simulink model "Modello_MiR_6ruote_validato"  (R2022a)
settings: Solver=VariableStepAuto  StartTime=0.0  StopTime=time_s(end,1)  RelTol=1e-3
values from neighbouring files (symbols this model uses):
  a = 0.250    (= 0.25)    [Modello_MiR_6ruote_validato_script.m]    (also in Modello_MiR_2ruote_script.m; Modello_MiR_6ruote_script.m; Modello_MiR_UR_script.m)
  a1 = 0.18265    [Modello_MiR_6ruote_validato_script.m]    (also in Modello_MiR_2ruote_script.m = deg2rad(5); Modello_MiR_6ruote_script.m = deg2rad(5); Modello_MiR_UR_script.m; UR_DHtable_e.m = 0)
  a2 = 0.40857    [Modello_MiR_6ruote_validato_script.m]    (also in Modello_MiR_2ruote_script.m = deg2rad(25); Modello_MiR_6ruote_script.m = deg2rad(25); Modello_MiR_UR_script.m; UR_DHtable_e.m = 612)
  Att_C1 = 0.01    [Modello_MiR_6ruote_validato_script.m]    (also in Modello_MiR_UR_script.m)
  Att_C2 = 0.01    [Modello_MiR_6ruote_validato_script.m]    (also in Modello_MiR_UR_script.m)
  Att_C5 = 0.01    [Modello_MiR_6ruote_validato_script.m]    (also in Modello_MiR_UR_script.m)
  Att_C6 = 0.01    [Modello_MiR_6ruote_validato_script.m]    (also in Modello_MiR_UR_script.m)
  b = 0.1875    [Modello_MiR_6ruote_validato_script.m]    (also in Modello_MiR_2ruote_script.m; Modello_MiR_6ruote_script.m; Modello_MiR_UR_script.m)
  b_caster = 0.07    [Modello_MiR_6ruote_validato_script.m]    (also in Modello_MiR_2ruote_script.m; Modello_MiR_6ruote_script.m; Modello_MiR_UR_script.m)
  bd = 0.205    [Modello_MiR_6ruote_validato_script.m]    (also in Modello_MiR_2ruote_script.m; Modello_MiR_6ruote_script.m; Modello_MiR_UR_script.m)
  F23fun = @(u) (mv*9.801/4)-(mv*h*u(5)+(mv*9.801/4)*(2*a-b_caster*(cos(u(1))+cos(u(2)))))/(4*a-b_caster*(cos(u(1))+cos(u(2)))+b_caster*(cos(u(3))+cos(u(4))))    [Modello_MiR_6ruote_validato_script.m]    (also in Modello_MiR_6ruote_script.m = @(u) (mv*9.801/4)-u(7))
  F43fun = @(u) (1/(2*bd))*(mv*u(6)*h+((mv*h*u(5)+(mv*9.801/4)*(2*a-b_caster*(cos(u(1))+cos(u(2)))))/(4*a-b_caster*(cos(u(1))+cos(u(2)))+b_caster*(cos(u(3))+cos(u(4)))))*(2*bd-b_caster*(sin(u(3))+sin(u(4))))+((mv*9.801/4)-(mv*h*u(5)+(mv*9.801/4)*(2*a-b_caster*(cos(u(1))+cos(u(2)))))/(4*a-b_caster*(cos(u(1))+cos(u(2)))+b_caster*(cos(u(3))+cos(u(4)))))*(2*bd-b_caster*(sin(u(1))+sin(u(2)))))    [Modello_MiR_6ruote_validato_script.m]    (also in Modello_MiR_6ruote_script.m = @(u) (1/(2*bd))*(mv*u(6)*h+u(7)*(2*bd-b_caster*(sin(u(3))+si)
  F63fun = @(u) (mv*h*u(5)+(mv*9.801/4)*(2*a-b_caster*(cos(u(1))+cos(u(2)))))/(4*a-b_caster*(cos(u(1))+cos(u(2)))+b_caster*(cos(u(3))+cos(u(4))))    [Modello_MiR_6ruote_validato_script.m]    (also in Modello_MiR_6ruote_script.m)
  f_c = 0.29564    [Modello_MiR_6ruote_validato_script.m]    (also in Modello_MiR_UR_script.m)
  f_d3 = 0.35846    [Modello_MiR_6ruote_validato_script.m]    (also in Modello_MiR_UR_script.m)
  f_d4 = 0.2333    [Modello_MiR_6ruote_validato_script.m]    (also in Modello_MiR_UR_script.m)
  fa_c = 0.27474    [Modello_MiR_6ruote_validato_script.m]    (also in Modello_MiR_UR_script.m)
  fa_d3 = 0.3694    [Modello_MiR_6ruote_validato_script.m]    (also in Modello_MiR_UR_script.m)
  fa_d4 = 0.28065    [Modello_MiR_6ruote_validato_script.m]    (also in Modello_MiR_UR_script.m)
  fm_fun = @(u) (u <= -am2 || u >= am2) * 0 + (u > -am2 && u <= -am1) * (- u* Mza/(am2 -am1) - Mza* am2/(am2 -am1)) +           + (u > -am1 && u <= am1) * (Mza * u / am1) + (u > am1 && u < am2) * (Mza * u /(am1 -am2) - Mza * am2 /(am1 - am2))    [Modello_MiR_6ruote_validato_script.m]    (also in Modello_MiR_6ruote_script.m = @(u) (u <= -am2 | u >= am2)*0 + (u > -am2 && u <= -am1)*(- u; Modello_MiR_UR_script.m)
  Icw_1 = 1/2 * mcw * rc^2    (= 0.002004225735)    [Modello_MiR_6ruote_validato_script.m]    (also in Modello_MiR_2ruote_script.m; Modello_MiR_6ruote_script.m; Modello_MiR_UR_script.m)
  Icw_2 = 1/12 * mcw * ec^2 + 1/4 * mcw * rc^2    (= 0.00104098243873)    [Modello_MiR_6ruote_validato_script.m]    (also in Modello_MiR_2ruote_script.m; Modello_MiR_6ruote_script.m; Modello_MiR_UR_script.m)
  Idw_1 = 1/2 * mdw * rd^2    (= 0.00551836278784)    [Modello_MiR_6ruote_validato_script.m]    (also in Modello_MiR_2ruote_script.m; Transfer_Function_Gol_Gcl.m = Inertia_vect(jj,1); Modello_MiR_6ruote_script.m; Modello_MiR_UR_script.m)
  iMax = 20.7*1.1    (= 22.77)    [Modello_MiR_6ruote_validato_script.m]    (also in Modello_MiR_2ruote_script.m; Modello_MiR_6ruote_script.m; Modello_MiR_UR_script.m)
  Iv = mv * (l^2 + w^2)  / 12    (= 8.95033333333)    [Modello_MiR_6ruote_validato_script.m]    (also in Modello_MiR_2ruote_script.m = 6.75343333333; Modello_MiR_6ruote_script.m = 6.75343333333; Modello_MiR_UR_script.m = 6.75343333333)
  Kc = 0.15    [Modello_MiR_6ruote_validato_script.m]    (also in Modello_MiR_2ruote_script.m; Modello_MiR_6ruote_script.m; Modello_MiR_UR_script.m)
  Ki_i = 1    [Modello_MiR_6ruote_validato_script.m]    (also in Modello_MiR_2ruote_script.m; Modello_MiR_6ruote_script.m; Modello_MiR_UR_script.m)
  Ki_v = 1    [Modello_MiR_6ruote_validato_script.m]    (also in Modello_MiR_2ruote_script.m; Modello_MiR_6ruote_script.m; Modello_MiR_UR_script.m)
  kk = 0.00005    (= 5e-05)    [Modello_MiR_6ruote_validato_script.m]    (also in Modello_MiR_2ruote_script.m; Modello_MiR_6ruote_script.m; Modello_MiR_UR_script.m)
  Kp_i = 5    [Modello_MiR_6ruote_validato_script.m]    (also in Modello_MiR_2ruote_script.m; Modello_MiR_6ruote_script.m; Modello_MiR_UR_script.m)
  Kp_v = 5    [Modello_MiR_6ruote_validato_script.m]    (also in Modello_MiR_2ruote_script.m; Modello_MiR_6ruote_script.m; Modello_MiR_UR_script.m)
  kv = 1.5e-6    (= 1.5e-06)    [Modello_MiR_6ruote_validato_script.m]    (also in Modello_MiR_2ruote_script.m; Modello_MiR_6ruote_script.m; Modello_MiR_UR_script.m)
  L = R * tauE    (= 0.00181134822805)    [Modello_MiR_6ruote_validato_script.m]    (also in Modello_MiR_2ruote_script.m; Modello_MiR_6ruote_script.m; Modello_MiR_UR_script.m)
  mcw = rc^2 * pi * ec * rhopoliu + 1    (= 1.02616357632)    [Modello_MiR_6ruote_validato_script.m]    (also in Modello_MiR_2ruote_script.m; Modello_MiR_6ruote_script.m; Modello_MiR_UR_script.m)
  mv = 110    [Modello_MiR_6ruote_validato_script.m]    (also in Modello_MiR_2ruote_script.m = 83; Modello_MiR_6ruote_script.m = 83; Modello_MiR_UR_script.m = 83)
  Phi1_start = psi_mir(1,1)    [Modello_MiR_6ruote_validato_script.m]    (also in Modello_MiR_UR_script.m)
  Phi2_start = psi_mir(1,1)    [Modello_MiR_6ruote_validato_script.m]    (also in Modello_MiR_UR_script.m)
  Phi5_start = psi_mir(1,1)    [Modello_MiR_6ruote_validato_script.m]    (also in Modello_MiR_UR_script.m)
  Phi6_start = psi_mir(1,1)    [Modello_MiR_6ruote_validato_script.m]    (also in Modello_MiR_UR_script.m)
  Psi_start = psi_mir(1,1)    [Modello_MiR_6ruote_validato_script.m]    (also in Modello_MiR_6ruote_script.m = 1.57079632679; Modello_MiR_UR_script.m)
  R = velMax * TorqueMax / (iMax)^2    (= 1.81134822805)    [Modello_MiR_6ruote_validato_script.m]    (also in Modello_MiR_2ruote_script.m; Modello_MiR_6ruote_script.m; Modello_MiR_UR_script.m)
  rap_rid = 10.167    [Modello_MiR_6ruote_validato_script.m]    (also in Modello_MiR_2ruote_script.m; Modello_MiR_6ruote_script.m; Modello_MiR_UR_script.m)
  rc = 0.125/2    (= 0.0625)    [Modello_MiR_6ruote_validato_script.m]    (also in Modello_MiR_2ruote_script.m; Modello_MiR_6ruote_script.m; Modello_MiR_UR_script.m)
  rd = 0.1    [Modello_MiR_6ruote_validato_script.m]    (also in Modello_MiR_2ruote_script.m; Modello_MiR_6ruote_script.m; Modello_MiR_UR_script.m)
  s1 = 0.18987    [Modello_MiR_6ruote_validato_script.m]    (also in Modello_MiR_2ruote_script.m = 0.2; Modello_MiR_6ruote_script.m = 0.2; Modello_MiR_UR_script.m)
  s2 = 0.99533    [Modello_MiR_6ruote_validato_script.m]    (also in Modello_MiR_2ruote_script.m = 0.8; Modello_MiR_6ruote_script.m = 0.8; Modello_MiR_UR_script.m)
  Sx = spline(x ,fl_fun(x),zx)    [Modello_MiR_6ruote_script.m]
  Sy = spline(x ,ft_fun(x),zy)    [Modello_MiR_6ruote_script.m]
  VaMax = Kc * velMax    (= 41.2443991527)    [Modello_MiR_6ruote_validato_script.m]    (also in Modello_MiR_2ruote_script.m; Modello_MiR_6ruote_script.m; Modello_MiR_UR_script.m)
  X_start = traj(1,1)    [Modello_MiR_6ruote_validato_script.m]    (also in Modello_MiR_2ruote_script.m = input('Inserire coordinata x iniziale'); Modello_MiR_6ruote_script.m = input('Inserire coordinata x iniziale'); Modello_MiR_UR_script.m)
  Y_start = traj(1,2)    [Modello_MiR_6ruote_validato_script.m]    (also in Modello_MiR_2ruote_script.m = input('Inserire coordinata y iniziale'); Modello_MiR_6ruote_script.m = input('Inserire coordinata y iniziale'); Modello_MiR_UR_script.m)
undefined symbols (not defined in the file or in its folder): z
libraries: slpidlib x4
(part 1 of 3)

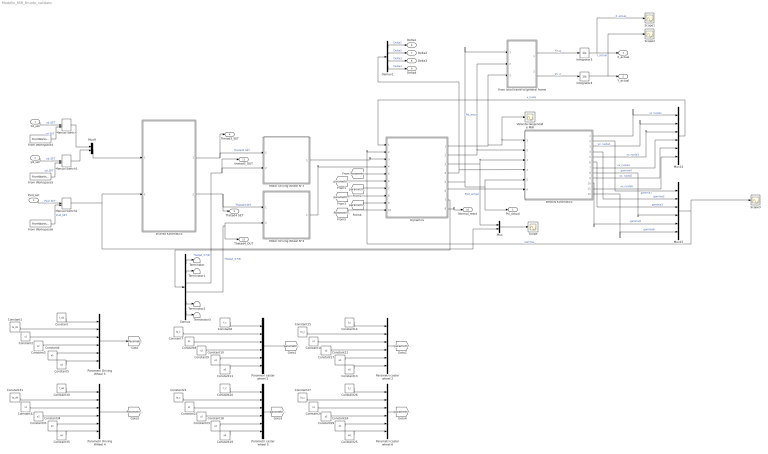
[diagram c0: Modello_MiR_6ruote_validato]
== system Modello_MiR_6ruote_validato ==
  xd_set : Inport
  yd_set : Inport  Port=2
  Psid_set : Inport  Port=3
  " Wheels Kinematics" : Subsystem
  Constant : Constant  Value=f_d3
  Constant1 : Constant  Value=fa_d3
  Constant{4,10,12,18,24,34} (6 alike) : Constant  Value=a1
  Constant{5,11,13,19,25,35} (6 alike) : Constant  Value=a2
  Constant{6,14,20,26} (4 alike) : Constant  Value=f_c
  Constant{7,15,21,27} (4 alike) : Constant  Value=fa_c
  Constant{2,8,16,22,28,32} (6 alike) : Constant  Value=s1
  Constant{3,9,17,23,29,33} (6 alike) : Constant  Value=s2
  Constant30 : Constant  Value=f_d4
  Constant31 : Constant  Value=fa_d4
  Demux : Demux  Outputs=6
  Demux1 : Demux
  Dynamics : Subsystem
  From Workspace4 : FromWorkspace  VariableName=[time_v xd_set]
  From Workspace5 : FromWorkspace  VariableName=[time_v yd_set]
  From Workspace6 : FromWorkspace  VariableName=[ time_v psid_set]
  From local frame to general frame : Subsystem
  Integrator3 : Integrator  InitialCondition=X_start
  Integrator4 : Integrator  InitialCondition=Y_start
  Inverse Kinematics : Subsystem
  Manual Switch : ManualSwitch  CurrentSetting=0
  Manual Switch1 : ManualSwitch  CurrentSetting=0
  Manual Switch2 : ManualSwitch  CurrentSetting=0
  Motor Driving Wheel N°3 : Subsystem
  Motor Driving Wheel N°4 : Subsystem
  Mux : Mux  Inputs=2
  Mux14 : Mux  Inputs=6
  Mux15 : Mux  Inputs=6
  Mux9 : Mux  Inputs=2
  Parametri Driving WHeel 4 : Mux  Inputs=6
  Parametri Driving Wheel 3 : Mux  Inputs=6
  "Parametri caster wheel 1 " : Mux  Inputs=6
  Parametri caster wheel 2 : Mux  Inputs=6
  Parametri caster wheel 5 : Mux  Inputs=6
  Parametri caster wheel 6 : Mux  Inputs=6
  Scope{,1..3} (4 alike) : Scope
  Terminator{,1..3} (4 alike) : Terminator
  Velocità tangenziale MIR : Scope
  Psi_actual : Outport
  Y_actual : Outport  Port=2
  X_actual : Outport  Port=3
  Thetad3_SET : Outport  Port=4
  Thetad4 SET : Outport  Port=5
  Delta1 : Outport  Port=6
  Delta2 : Outport  Port=7
  Delta3 : Outport  Port=8
  Delta4 : Outport  Port=9
  Normal_react : Outport  Port=10
  thetad3_OUT : Outport  Port=11
  Thetad4_OUT : Outport  Port=12
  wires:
  From local frame to general frame/2(Vy_g) -> Integrator4/1  "Vy_g"
  Dynamics/6(Phid) -> " Wheels Kinematics"/6(Phid)
  " Wheels Kinematics"/9(vx_ruota5) -> Mux14/5  "vx_ruota5"
  " Wheels Kinematics"/4(gamma2) -> Mux15/2  "gamma2"
  " Wheels Kinematics"/11(vx_ruota6) -> Mux14/6  "vx_ruota6"
  " Wheels Kinematics"/12(gamma6) -> Mux15/6  "gamma6"
  " Wheels Kinematics"/10(gamma5) -> Mux15/5  "gamma5"
  " Wheels Kinematics"/8(gamma4) -> Mux15/4  "gamma4"
  " Wheels Kinematics"/3(vx_ruota2) -> Mux14/2  "vx_ruota2"
  Dynamics/7(Thetad) -> Demux/1
  Motor Driving Wheel N°3/1(Cm_L) -> Dynamics/3(Cm3)
  From Workspace6/1 -> Manual Switch2/2  "Psid_SET"
  Mux/1 -> Scope/1
  Dynamics/4(Delta) -> Demux1/1, " Wheels Kinematics"/4(Delta)
  Dynamics/5(Psi) -> From local frame to general frame/1(Psi), Psi_actual/1, " Wheels Kinematics"/5(Psi)  "Psi_actual"
  " Wheels Kinematics"/7(vx_ruota4) -> Mux14/4  "vx_ruota4"
  Demux/6 -> Terminator3/1
  Mux15/1 -> Scope3/1, Dynamics/2(gamma)  "gamma"
  " Wheels Kinematics"/2(gamma1) -> Mux15/1  "gamma1"
  Demux/5 -> Terminator2/1
  Integrator4/1 -> Scope2/1, Y_actual/1  "Y_actual"
  Mux9/1 -> Inverse Kinematics/1(vSet)
  Dynamics/1(xd) -> From local frame to general frame/3(Vx), Velocità tangenziale MIR/1, " Wheels Kinematics"/1(xd)
  " Wheels Kinematics"/5(vx_ruota3) -> Mux14/3  "vx_ruota3"
  Dynamics/3(Psid) -> " Wheels Kinematics"/3(Psid), Mux/1  "Psid_actual"
  " Wheels Kinematics"/6(gamma3) -> Mux15/3  "gamma3"
  Integrator3/1 -> Scope1/1, X_actual/1  "X_actual"
  Inverse Kinematics/2(ThetaDotR) -> Thetad4 SET/1, Motor Driving Wheel N°4/1(ThetadR_SET)  "Thetad4 SET"
  Demux/4 -> Thetad4_OUT/1, Motor Driving Wheel N°4/2(ThetadR_FB)  "Thetad_4 F/B"
  Demux/2 -> Terminator1/1
  From local frame to general frame/1(Vx_g) -> Integrator3/1  "Vx_g"
  Mux14/1 -> Dynamics/1(vx_ruote)  "v_ruote"
  Dynamics/2(yd) -> From local frame to general frame/2(Vy), " Wheels Kinematics"/2(yd)
  Demux/1 -> Terminator/1
  " Wheels Kinematics"/1(vx_ruota1) -> Mux14/1  "vx_ruota1"
  Inverse Kinematics/1(ThetaDotL) -> Thetad3_SET/1, Motor Driving Wheel N°3/1(ThetadL_SET)  "Thetad3 SET"
  From Workspace5/1 -> Manual Switch1/2  "yd_SET"
  Motor Driving Wheel N°4/1(Cm_R) -> Dynamics/4(Cm4)
  Demux/3 -> thetad3_OUT/1, Motor Driving Wheel N°3/2(ThetadL_FB)  "Thetad_3 F/B"
  From Workspace4/1 -> Manual Switch/2  "xd_SET"
  Demux1/1 -> Delta1/1  "Delta1"
  Demux1/2 -> Delta2/1  "Delta2"
  Demux1/3 -> Delta3/1  "Delta3"
  Demux1/4 -> Delta4/1  "Delta4"
  Dynamics/8(Normal_react) -> Normal_react/1
  Parametri Driving Wheel 3/1 -> [Parametri]
  [Parametri] -> Dynamics/5(parametri_dw3)
  Constant/1 -> Parametri Driving Wheel 3/1
  Constant5/1 -> Parametri Driving Wheel 3/6
  Constant4/1 -> Parametri Driving Wheel 3/5
  Constant3/1 -> Parametri Driving Wheel 3/4
  Constant2/1 -> Parametri Driving Wheel 3/3
  Constant1/1 -> Parametri Driving Wheel 3/2
  xd_set/1 -> Manual Switch/1  "xd_SET"
  Manual Switch/1 -> Mux9/1
  yd_set/1 -> Manual Switch1/1  "yd_SET"
  Manual Switch1/1 -> Mux9/2
  Psid_set/1 -> Manual Switch2/1  "Psid_SET"
  Manual Switch2/1 -> Mux/2, Inverse Kinematics/2(psiDotSet)
  Constant10/1 -> "Parametri caster wheel 1 "/5
  Constant8/1 -> "Parametri caster wheel 1 "/3
  Constant9/1 -> "Parametri caster wheel 1 "/4
  Constant7/1 -> "Parametri caster wheel 1 "/2
  Constant11/1 -> "Parametri caster wheel 1 "/6
  Constant6/1 -> "Parametri caster wheel 1 "/1
  "Parametri caster wheel 1 "/1 -> [parametri_cw1]
  Constant12/1 -> Parametri caster wheel 2/5
  Constant17/1 -> Parametri caster wheel 2/4
  Constant16/1 -> Parametri caster wheel 2/3
  Constant13/1 -> Parametri caster wheel 2/6
  Constant15/1 -> Parametri caster wheel 2/2
  Constant14/1 -> Parametri caster wheel 2/1
  Parametri caster wheel 2/1 -> [parametri_cw2]
  Constant21/1 -> Parametri caster wheel 5/2
  Constant22/1 -> Parametri caster wheel 5/3
  Constant20/1 -> Parametri caster wheel 5/1
  Constant19/1 -> Parametri caster wheel 5/6
  Constant18/1 -> Parametri caster wheel 5/5
  Constant23/1 -> Parametri caster wheel 5/4
  Parametri caster wheel 5/1 -> [parametri_cw5]
  Constant27/1 -> Parametri caster wheel 6/2
  Constant28/1 -> Parametri caster wheel 6/3
  Constant26/1 -> Parametri caster wheel 6/1
  Constant25/1 -> Parametri caster wheel 6/6
  Constant24/1 -> Parametri caster wheel 6/5
  Constant29/1 -> Parametri caster wheel 6/4
  Parametri caster wheel 6/1 -> [parametri_cw6]
  [parametri_cw1] -> Dynamics/6(parametri_cw1)
  [parametri_cw2] -> Dynamics/7(parametri_cw2)
  [parametri_cw5] -> Dynamics/8(parametri_cw5)
  [parametri_cw6] -> Dynamics/9(parametri_cw6)
  Constant35/1 -> Parametri Driving WHeel 4/6
  Constant34/1 -> Parametri Driving WHeel 4/5
  Constant33/1 -> Parametri Driving WHeel 4/4
  Constant32/1 -> Parametri Driving WHeel 4/3
  Constant31/1 -> Parametri Driving WHeel 4/2
  Parametri Driving WHeel 4/1 -> [Parametri_dw4]
  Constant30/1 -> Parametri Driving WHeel 4/1
  [Parametri_dw4] -> Dynamics/10(parametri_dw4)

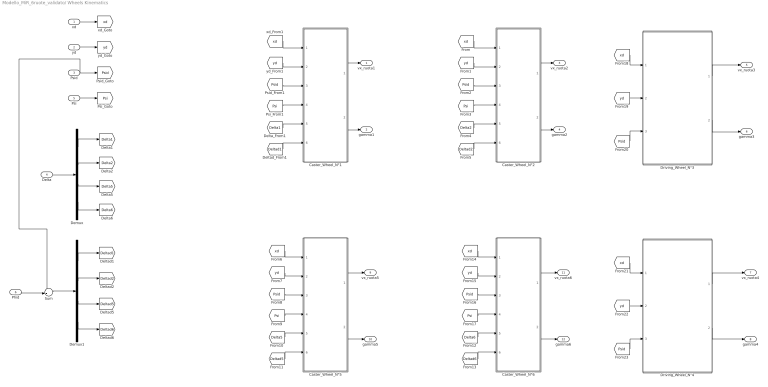
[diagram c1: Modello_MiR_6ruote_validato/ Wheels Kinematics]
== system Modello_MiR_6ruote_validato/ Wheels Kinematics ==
  xd : Inport
  yd : Inport  Port=2
  Psid : Inport  Port=3
  Delta : Inport  Port=4
  Psi : Inport  Port=5
  Phid : Inport  Port=6
  Caster_Wheel_N°1 : Subsystem
  Caster_Wheel_N°2 : Subsystem
  Caster_Wheel_N°5 : Subsystem
  Caster_Wheel_N°6 : Subsystem
  Demux : Demux
  Demux1 : Demux
  Driving_Wheel_N°3 : Subsystem
  Driving_Wheel_N°4 : Subsystem
  Sum : Sum  Inputs=-+|
  vx_ruota1 : Outport
  gamma1 : Outport  Port=2
  vx_ruota2 : Outport  Port=3
  gamma2 : Outport  Port=4
  vx_ruota3 : Outport  Port=5
  gamma3 : Outport  Port=6
  vx_ruota4 : Outport  Port=7
  gamma4 : Outport  Port=8
  vx_ruota5 : Outport  Port=9
  gamma5 : Outport  Port=10
  vx_ruota6 : Outport  Port=11
  gamma6 : Outport  Port=12
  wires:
  xd/1 -> [xd]
  yd/1 -> [yd]
  Psid/1 -> [Psid], Sum/1
  Delta/1 -> Demux/1
  Demux/1 -> [Delta1]
  Demux/2 -> [Delta2]
  Demux/3 -> [Delta5]
  Demux/4 -> [Delta6]
  Psi/1 -> [Psi]
  Phid/1 -> Sum/2
  Demux1/1 -> [Deltad1]
  Demux1/2 -> [Deltad2]
  Demux1/3 -> [Deltad5]
  Demux1/4 -> [Deltad6]
  [xd] -> Caster_Wheel_N°1/1(xd_From1)
  [yd] -> Caster_Wheel_N°1/2(yd_From1)
  [Psid] -> Caster_Wheel_N°1/3(Psid_From1)
  [Psi] -> Caster_Wheel_N°1/4(Psi_From1)
  [Delta1] -> Caster_Wheel_N°1/5(Delta_From1)
  [Deltad1] -> Caster_Wheel_N°1/6(Deltad_From1)
  Caster_Wheel_N°1/1(vx_ruota1) -> vx_ruota1/1
  Caster_Wheel_N°1/2(gamma1) -> gamma1/1
  [yd] -> Caster_Wheel_N°2/2(yd_From1)
  [Psi] -> Caster_Wheel_N°2/4(Psi_From1)
  [Psid] -> Caster_Wheel_N°2/3(Psid_From1)
  [xd] -> Caster_Wheel_N°2/1(xd_From1)
  [Deltad2] -> Caster_Wheel_N°2/6(Deltad_From2)
  Caster_Wheel_N°2/2(gamma2) -> gamma2/1
  [Delta2] -> Caster_Wheel_N°2/5(Delta_From2)
  Caster_Wheel_N°2/1(vx_ruota2) -> vx_ruota2/1
  [xd] -> Caster_Wheel_N°5/1(xd_From1)
  Caster_Wheel_N°5/2(gamma5) -> gamma5/1
  Caster_Wheel_N°5/1(vx_ruota5) -> vx_ruota5/1
  [Psid] -> Caster_Wheel_N°5/3(Psid_From1)
  [Deltad5] -> Caster_Wheel_N°5/6(Deltad_From5)
  [yd] -> Caster_Wheel_N°5/2(yd_From1)
  [Delta5] -> Caster_Wheel_N°5/5(Delta_From5)
  [Psi] -> Caster_Wheel_N°5/4(Psi_From1)
  Caster_Wheel_N°6/1(vx_ruota6) -> vx_ruota6/1
  [yd] -> Caster_Wheel_N°6/2(yd_From1)
  [Psid] -> Caster_Wheel_N°6/3(Psid_From1)
  [Psi] -> Caster_Wheel_N°6/4(Psi_From1)
  Caster_Wheel_N°6/2(gamma6) -> gamma6/1
  [xd] -> Caster_Wheel_N°6/1(xd_From1)
  [Delta6] -> Caster_Wheel_N°6/5(Delta_From6)
  [Deltad6] -> Caster_Wheel_N°6/6(Deltad_From6)
  [xd] -> Driving_Wheel_N°3/1(xd_From1)
  [yd] -> Driving_Wheel_N°3/2(yd_From1)
  [Psid] -> Driving_Wheel_N°3/3(Psid_From1)
  [xd] -> Driving_Wheel_N°4/1(xd_From1)
  [yd] -> Driving_Wheel_N°4/2(yd_From1)
  [Psid] -> Driving_Wheel_N°4/3(Psid_From1)
  Driving_Wheel_N°3/1(vx_ruota3) -> vx_ruota3/1
  Driving_Wheel_N°3/2(gamma3) -> gamma3/1
  Driving_Wheel_N°4/1(vx_ruota4) -> vx_ruota4/1
  Driving_Wheel_N°4/2(gamma4) -> gamma4/1
  Sum/1 -> Demux1/1

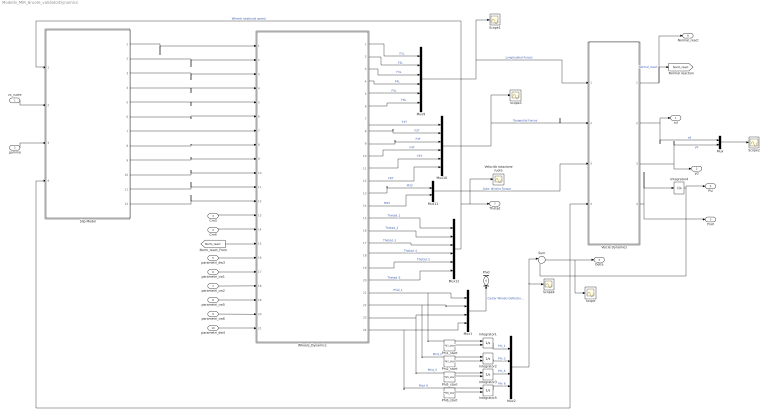
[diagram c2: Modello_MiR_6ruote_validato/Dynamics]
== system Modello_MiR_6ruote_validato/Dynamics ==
  vx_ruote : Inport
  gamma : Inport  Port=2
  Cm3 : Inport  Port=3
  Cm4 : Inport  Port=4
  parametri_dw3 : Inport  Port=5
  parametri_cw1 : Inport  Port=6
  parametri_cw2 : Inport  Port=7
  parametri_cw5 : Inport  Port=8
  parametri_cw6 : Inport  Port=9
  parametri_dw4 : Inport  Port=10
  Integrator{1..3,5} (4 alike) : Integrator  InitialConditionSource=external
  Integrator4 : Integrator  InitialCondition=Psi_start
  Mux : Mux  Inputs=2
  Mux1 : Mux
  Mux10 : Mux  Inputs=6
  Mux11 : Mux  Inputs=2
  Mux12 : Mux  Inputs=6
  Mux2 : Mux
  Mux9 : Mux  Inputs=6
  Phi1_start : Constant  Value=Phi1_start
  Phi2_start : Constant  Value=Phi2_start
  Phi5_start : Constant  Value=Phi5_start
  Phi6_start : Constant  Value=Phi6_start
  Scope{,1..4} (5 alike) : Scope
  Slip Model : Subsystem
  Sum : Sum  Inputs=|+-
  Veicle Dynamics : Subsystem
  Velocità rotazione ruote : Scope
  Wheels_Dynamics : Subsystem
  xd : Outport  PortDimensions=1
  yd : Outport  Port=2  PortDimensions=1
  Psid : Outport  Port=3  PortDimensions=1
  Delta : Outport  Port=4
  Psi : Outport  Port=5  PortDimensions=1
  Phid : Outport  Port=6
  Thetad : Outport  Port=7
  Normal_react : Outport  Port=8
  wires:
  Wheels_Dynamics/14(M43) -> Mux11/2  "M43"
  Wheels_Dynamics/23(Phid_5) -> Integrator3/1, Mux1/3  "Phid_5"
  Wheels_Dynamics/8(F2T) -> Mux10/2  "F2T"
  Wheels_Dynamics/12(F6T) -> Mux10/6  "F6T"
  Wheels_Dynamics/19(Thetad_5) -> Mux12/5  "Thetad_5"
  Wheels_Dynamics/18(Thetad_4) -> Mux12/4  "Thetad_4"
  Slip Model/1(Sigma1) -> Wheels_Dynamics/1(Sigma1)
  Wheels_Dynamics/2(F2L) -> Mux9/2  "F2L"
  Wheels_Dynamics/4(F4L) -> Mux9/4  "F4L"
  Wheels_Dynamics/3(F3L) -> Mux9/3  "F3L"
  Veicle Dynamics/4(Psid) -> Psid/1, Integrator4/1
  Wheels_Dynamics/1(F1L) -> Mux9/1  "F1L"
  Slip Model/3(Sigma3) -> Wheels_Dynamics/3(Sigma3)
  Slip Model/11(alpha5) -> Wheels_Dynamics/11(alpha5)
  Wheels_Dynamics/5(F5L) -> Mux9/5  "F5L"
  Slip Model/9(alpha3) -> Wheels_Dynamics/9(alpha3)
  Wheels_Dynamics/16(Thetad_2) -> Mux12/2  "Thetad_2"
  Mux1/1 -> Phid/1  "Caster Wheels Deflection Velocity"
  Cm3/1 -> Wheels_Dynamics/13(Cm3)
  Mux11/1 -> Veicle Dynamics/3(M)  "Auto_allining Torque"
  Wheels_Dynamics/10(F4T) -> Mux10/4  "F4T"
  Wheels_Dynamics/13(M33) -> Mux11/1  "M33"
  Mux12/1 -> Slip Model/1(Thetad_ruote), Velocità rotazione ruote/1, Thetad/1  "Wheels rotational speed"
  Mux10/1 -> Scope3/1, Veicle Dynamics/2(FT)  "Tangential Forces"
  Slip Model/5(Sigma5) -> Wheels_Dynamics/5(Sigma5)
  Wheels_Dynamics/21(Phid_1) -> Integrator1/1, Mux1/1  "Phid_1"
  Wheels_Dynamics/6(F6L) -> Mux9/6  "F6L"
  Wheels_Dynamics/17(Thetad_3) -> Mux12/3  "Thetad_3"
  Wheels_Dynamics/15(Thetad_1) -> Mux12/1  "Thetad_1"
  Wheels_Dynamics/24(Phid_6) -> Integrator5/1, Mux1/4  "Phid_6"
  Wheels_Dynamics/11(F5T) -> Mux10/5  "F5T"
  Wheels_Dynamics/9(F3T) -> Mux10/3  "F3T"
  Wheels_Dynamics/7(F1T) -> Mux10/1  "F1T"
  Wheels_Dynamics/22(Phid_2) -> Integrator2/1, Mux1/2  "Phid_2"
  Veicle Dynamics/1(Normal_react) -> Normal_react/1, [Norm_react]  "Normal_react"
  Veicle Dynamics/2(xd) -> Mux/1, xd/1  "xd"
  Mux2/1 -> Sum/1, Scope4/1
  Wheels_Dynamics/20(Thetad_6) -> Mux12/6  "Thetad_6"
  Slip Model/8(alpha2) -> Wheels_Dynamics/8(alpha2)
  Integrator4/1 -> Psi/1, Sum/2
  [Norm_react] -> Wheels_Dynamics/15(Normal_React)
  Veicle Dynamics/3(yd) -> Mux/2, yd/1  "yd"
  Mux9/1 -> Scope1/1, Veicle Dynamics/1(FL)  "Longitudinal Forces"
  Slip Model/4(Sigma4) -> Wheels_Dynamics/4(Sigma4)
  Slip Model/10(alpha4) -> Wheels_Dynamics/10(alpha4)
  Slip Model/12(alpha6) -> Wheels_Dynamics/12(alpha6)
  Slip Model/7(alpha1) -> Wheels_Dynamics/7(alpha1)
  Slip Model/2(Sigma2) -> Wheels_Dynamics/2(Sigma2)
  Slip Model/6(Sigma6) -> Wheels_Dynamics/6(Sigma6)
  vx_ruote/1 -> Slip Model/2(vx_ruote)
  gamma/1 -> Slip Model/3(gamma)
  Cm4/1 -> Wheels_Dynamics/14(Cm4)
  Mux/1 -> Scope2/1
  Sum/1 -> Slip Model/4(Delta), Scope/1, Delta/1, Veicle Dynamics/4(Delta)
  parametri_dw3/1 -> Wheels_Dynamics/16(parametri_dw3)
  parametri_cw1/1 -> Wheels_Dynamics/17(parametri_cw1)
  parametri_cw2/1 -> Wheels_Dynamics/18(parametri_cw2)
  parametri_cw5/1 -> Wheels_Dynamics/19(parametri_cw5)
  parametri_cw6/1 -> Wheels_Dynamics/20(parametri_cw6)
  Integrator1/1 -> Mux2/1  "Phi_1"
  Integrator2/1 -> Mux2/2  "Phi_2"
  Integrator3/1 -> Mux2/3  "Phi_5"
  Integrator5/1 -> Mux2/4  "Phi_6"
  Phi1_start/1 -> Integrator1/2
  Phi2_start/1 -> Integrator2/2
  Phi5_start/1 -> Integrator3/2
  Phi6_start/1 -> Integrator5/2
  parametri_dw4/1 -> Wheels_Dynamics/21(parametri_dw4)

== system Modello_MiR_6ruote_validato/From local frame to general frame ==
  Psi : Inport
  Vy : Inport  Port=2
  Vx : Inport  Port=3
  Cos : Trigonometry  Operator=cos
  Product{,1..3} (4 alike) : Product
  Sin : Trigonometry
  Sum : Sum  Inputs=-+
  Sum1 : Sum  Inputs=|++
  Vx_g : Outport
  Vy_g : Outport  Port=2
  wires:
  Product/1 -> Sum/2
  Sin/1 -> Product2/2, Product1/2
  Product1/1 -> Sum/1
  Vx/1 -> Product2/1, Product/1
  Product2/1 -> Sum1/1
  Cos/1 -> Product3/1, Product/2
  Product3/1 -> Sum1/2
  Psi/1 -> Sin/1, Cos/1
  Vy/1 -> Product3/2, Product1/1
  Sum/1 -> Vx_g/1
  Sum1/1 -> Vy_g/1

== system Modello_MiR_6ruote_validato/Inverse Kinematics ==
  vSet : Inport
  psiDotSet : Inport  Port=2
  Demux : Demux  Outputs=2
  MATLAB Function : MATLAB Function  TreatAsAtomicUnit=on
  MATLAB Function1 : MATLAB Function  TreatAsAtomicUnit=on
  Scope1 : Scope
  Scope2 : Scope
  Terminator : Terminator
  ThetaDotL : Outport
  ThetaDotR : Outport  Port=2
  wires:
  vSet/1 -> Demux/1
  Demux/1 -> MATLAB Function1/1(xd_set), MATLAB Function/1(xd_set)  "xd_set"
  psiDotSet/1 -> MATLAB Function1/2(psid_set), MATLAB Function/2(psid_set)
  MATLAB Function/1(Thetad_DR_SET) -> Scope1/1, ThetaDotR/1
  MATLAB Function1/1(Thetad_DL_SET) -> Scope2/1, ThetaDotL/1
  Demux/2 -> Terminator/1  "yd_set"

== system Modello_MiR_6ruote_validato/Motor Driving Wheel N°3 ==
  ThetadL_SET : Inport
  ThetadL_FB : Inport  Port=2
  Gain : Gain  Gain=rap_rid
  Gain1 : Gain  Gain=rap_rid
  Subsystem : Subsystem
  Subsystem1 : Subsystem
  Cm_L : Outport
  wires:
  Subsystem/1(VaRif) -> Subsystem1/1(VaRif)
  Subsystem1/2(iFB) -> Subsystem/3(iFB)
  ThetadL_SET/1 -> Gain1/1
  ThetadL_FB/1 -> Gain/1
  Subsystem1/1(Torque Cm) -> Cm_L/1
  Gain/1 -> Subsystem1/2(Thetad_FB), Subsystem/2(Thetad_FB)
  Gain1/1 -> Subsystem/1(Thetad_SET)

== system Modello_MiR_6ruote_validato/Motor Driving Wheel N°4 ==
  ThetadR_SET : Inport
  ThetadR_FB : Inport  Port=2
  Gain : Gain  Gain=rap_rid
  Gain1 : Gain  Gain=rap_rid
  Subsystem : Subsystem
  Subsystem1 : Subsystem
  Cm_R : Outport
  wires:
  Subsystem1/2(iFB) -> Subsystem/3(iFB)
  ThetadR_SET/1 -> Gain1/1
  Subsystem/1(VaRif) -> Subsystem1/1(VaRif)
  ThetadR_FB/1 -> Gain/1
  Subsystem1/1(Torque Cm) -> Cm_R/1
  Gain/1 -> Subsystem1/2(Thetad_FB), Subsystem/2(Thetad_FB)
  Gain1/1 -> Subsystem/1(Thetad_SET)

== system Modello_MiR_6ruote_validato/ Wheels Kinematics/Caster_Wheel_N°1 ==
  xd_From1 : Inport
  yd_From1 : Inport  Port=2
  Psid_From1 : Inport  Port=3
  Psi_From1 : Inport  Port=4
  Delta_From1 : Inport  Port=5
  Deltad_From1 : Inport  Port=6
  Interpreted MATLAB Function : MATLABFcn  MATLABFcn=(u(1)^2+u(2)^2)^0.5
  Interpreted MATLAB Function2 : MATLABFcn  MATLABFcn=asin(u(2)/((u(1)^2+u(2)^2)^0.5+(1/cccc)*((u(1)^2+u(2)^2)==0)))
  Mux : Mux  Inputs=6
  Mux1 : Mux  Inputs=2
  xd_ruota1 : MATLABFcn  MATLABFcn=(u(6)+u(3))*b_caster*sin(u(5))+u(1)-u(3)*b
  yd_ruota1 : MATLABFcn  MATLABFcn=-(u(6)+u(3))*b_caster*cos(u(5))+u(2)+u(3)*a
  vx_ruota1 : Outport  PortDimensions=1
  gamma1 : Outport  Port=2  PortDimensions=1
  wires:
  Mux/1 -> xd_ruota1/1, yd_ruota1/1
  Mux1/1 -> Interpreted MATLAB Function/1, Interpreted MATLAB Function2/1
  yd_ruota1/1 -> Mux1/2  "yd_ruota1"
  yd_From1/1 -> Mux/2
  xd_ruota1/1 -> Mux1/1  "xd_ruota1"
  xd_From1/1 -> Mux/1
  Psid_From1/1 -> Mux/3
  Delta_From1/1 -> Mux/5
  Psi_From1/1 -> Mux/4
  Deltad_From1/1 -> Mux/6
  Interpreted MATLAB Function2/1 -> gamma1/1  "gamma1"
  Interpreted MATLAB Function/1 -> vx_ruota1/1  "vx_ruota1"

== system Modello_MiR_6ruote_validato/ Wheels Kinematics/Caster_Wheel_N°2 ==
  xd_From1 : Inport
  yd_From1 : Inport  Port=2
  Psid_From1 : Inport  Port=3
  Psi_From1 : Inport  Port=4
  Delta_From2 : Inport  Port=5
  Deltad_From2 : Inport  Port=6
  Interpreted MATLAB Function : MATLABFcn  MATLABFcn=(u(1)^2+u(2)^2)^0.5
  Interpreted MATLAB Function2 : MATLABFcn  MATLABFcn=asin(u(2)/((u(1)^2+u(2)^2)^0.5+(1/cccc)*((u(1)^2+u(2)^2)==0)))
  Mux : Mux  Inputs=6
  Mux1 : Mux  Inputs=2
  xd_ruota2 : MATLABFcn  MATLABFcn=(u(6)+u(3))*b_caster*sin(u(5))+u(1)+u(3)*b
  yd_ruota2 : MATLABFcn  MATLABFcn=-(u(6)+u(3))*b_caster*cos(u(5))+u(2)+u(3)*a
  vx_ruota2 : Outport  PortDimensions=1
  gamma2 : Outport  Port=2  PortDimensions=1
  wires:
  Mux/1 -> xd_ruota2/1, yd_ruota2/1
  Mux1/1 -> Interpreted MATLAB Function/1, Interpreted MATLAB Function2/1
  yd_ruota2/1 -> Mux1/2  "yd_ruota2"
  yd_From1/1 -> Mux/2
  xd_ruota2/1 -> Mux1/1  "xd_ruota2"
  xd_From1/1 -> Mux/1
  Psid_From1/1 -> Mux/3
  Delta_From2/1 -> Mux/5
  Psi_From1/1 -> Mux/4
  Deltad_From2/1 -> Mux/6
  Interpreted MATLAB Function2/1 -> gamma2/1  "gamma2"
  Interpreted MATLAB Function/1 -> vx_ruota2/1  "vx_ruota2"

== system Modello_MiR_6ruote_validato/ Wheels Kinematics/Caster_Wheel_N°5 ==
  xd_From1 : Inport
  yd_From1 : Inport  Port=2
  Psid_From1 : Inport  Port=3
  Psi_From1 : Inport  Port=4
  Delta_From5 : Inport  Port=5
  Deltad_From5 : Inport  Port=6
  Interpreted MATLAB Function : MATLABFcn  MATLABFcn=(u(1)^2+u(2)^2)^0.5
  Interpreted MATLAB Function2 : MATLABFcn  MATLABFcn=asin(u(2)/((u(1)^2+u(2)^2)^0.5+(1/cccc)*((u(1)^2+u(2)^2)==0)))
  Mux : Mux  Inputs=6
  Mux1 : Mux  Inputs=2
  xd_ruota5 : MATLABFcn  MATLABFcn=(u(6)+u(3))*b_caster*sin(u(5))+u(1)-u(3)*b
  yd_ruota5 : MATLABFcn  MATLABFcn=-(u(6)+u(3))*b_caster*cos(u(5))+u(2)-u(3)*a
  vx_ruota5 : Outport  PortDimensions=1
  gamma5 : Outport  Port=2  PortDimensions=1
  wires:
  Mux/1 -> xd_ruota5/1, yd_ruota5/1
  Mux1/1 -> Interpreted MATLAB Function/1, Interpreted MATLAB Function2/1
  yd_ruota5/1 -> Mux1/2  "yd_ruota5"
  yd_From1/1 -> Mux/2
  xd_ruota5/1 -> Mux1/1  "xd_ruota5"
  xd_From1/1 -> Mux/1
  Psid_From1/1 -> Mux/3
  Delta_From5/1 -> Mux/5
  Psi_From1/1 -> Mux/4
  Deltad_From5/1 -> Mux/6
  Interpreted MATLAB Function2/1 -> gamma5/1  "gamma5"
  Interpreted MATLAB Function/1 -> vx_ruota5/1  "v_ruota5"

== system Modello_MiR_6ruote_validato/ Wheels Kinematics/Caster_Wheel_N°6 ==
  xd_From1 : Inport
  yd_From1 : Inport  Port=2
  Psid_From1 : Inport  Port=3
  Psi_From1 : Inport  Port=4
  Delta_From6 : Inport  Port=5
  Deltad_From6 : Inport  Port=6
  Interpreted MATLAB Function : MATLABFcn  MATLABFcn=(u(1)^2+u(2)^2)^0.5
  Interpreted MATLAB Function2 : MATLABFcn  MATLABFcn=asin(u(2)/((u(1)^2+u(2)^2)^0.5+(1/cccc)*((u(1)^2+u(2)^2)==0)))
  Mux : Mux  Inputs=6
  Mux1 : Mux  Inputs=2
  xd_ruota6 : MATLABFcn  MATLABFcn=(u(6)+u(3))*b_caster*sin(u(5))+u(1)+u(3)*b
  yd_ruota6 : MATLABFcn  MATLABFcn=-(u(6)+u(3))*b_caster*cos(u(5))+u(2)-u(3)*a
  vx_ruota6 : Outport  PortDimensions=1
  gamma6 : Outport  Port=2  PortDimensions=1
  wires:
  Mux/1 -> xd_ruota6/1, yd_ruota6/1
  Mux1/1 -> Interpreted MATLAB Function/1, Interpreted MATLAB Function2/1
  yd_ruota6/1 -> Mux1/2  "yd_ruota6"
  yd_From1/1 -> Mux/2
  xd_ruota6/1 -> Mux1/1  "xd_ruota6"
  xd_From1/1 -> Mux/1
  Psid_From1/1 -> Mux/3
  Delta_From6/1 -> Mux/5
  Psi_From1/1 -> Mux/4
  Deltad_From6/1 -> Mux/6
  Interpreted MATLAB Function2/1 -> gamma6/1  "gamma6"
  Interpreted MATLAB Function/1 -> vx_ruota6/1  "v_ruota6"

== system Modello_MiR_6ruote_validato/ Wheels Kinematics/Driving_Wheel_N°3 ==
  xd_From1 : Inport
  yd_From1 : Inport  Port=2
  Psid_From1 : Inport  Port=3
  Interpreted MATLAB Function : MATLABFcn  MATLABFcn=u(1) - u(3)*bd
  Interpreted MATLAB Function1 : MATLABFcn  MATLABFcn=u(2)
  Interpreted MATLAB Function3 : MATLABFcn  MATLABFcn=asin(u(2)/((u(1)^2+u(2)^2)^0.5+(1/cccc)*((u(1)^2+u(2)^2)==0)))
  Mux : Mux  Inputs=3
  Mux1 : Mux  Inputs=2
  Scope1 : Scope
  vx_ruota3 : Outport  PortDimensions=1
  gamma3 : Outport  Port=2  PortDimensions=1
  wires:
  yd_From1/1 -> Mux/2
  xd_From1/1 -> Mux/1
  Psid_From1/1 -> Mux/3
  Mux/1 -> Interpreted MATLAB Function1/1, Interpreted MATLAB Function/1
  Interpreted MATLAB Function1/1 -> Mux1/2  "yd_ruota3"
  Interpreted MATLAB Function/1 -> vx_ruota3/1, Mux1/1  "xd_ruota3"
  Interpreted MATLAB Function3/1 -> gamma3/1  "gamma3"
  Mux1/1 -> Scope1/1, Interpreted MATLAB Function3/1

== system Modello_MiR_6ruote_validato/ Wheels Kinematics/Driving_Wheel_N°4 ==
  xd_From1 : Inport
  yd_From1 : Inport  Port=2
  Psid_From1 : Inport  Port=3
  Interpreted MATLAB Function : MATLABFcn  MATLABFcn=u(1) + u(3)*bd
  Interpreted MATLAB Function1 : MATLABFcn  MATLABFcn=u(2)
  Interpreted MATLAB Function3 : MATLABFcn  MATLABFcn=asin(u(2)/((u(1)^2+u(2)^2)^0.5+(1/cccc)*((u(1)^2+u(2)^2)==0)))
  Mux : Mux  Inputs=3
  Mux1 : Mux  Inputs=2
  Scope : Scope
  vx_ruota4 : Outport  PortDimensions=1
  gamma4 : Outport  Port=2  PortDimensions=1
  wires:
  yd_From1/1 -> Mux/2
  xd_From1/1 -> Mux/1
  Psid_From1/1 -> Mux/3
  Mux/1 -> Interpreted MATLAB Function1/1, Interpreted MATLAB Function/1
  Interpreted MATLAB Function1/1 -> Mux1/2  "yd_ruota4"
  Interpreted MATLAB Function/1 -> vx_ruota4/1, Mux1/1, Scope/1  "xd_ruota4"
  Mux1/1 -> Interpreted MATLAB Function3/1
  Interpreted MATLAB Function3/1 -> gamma4/1  "gamma4"

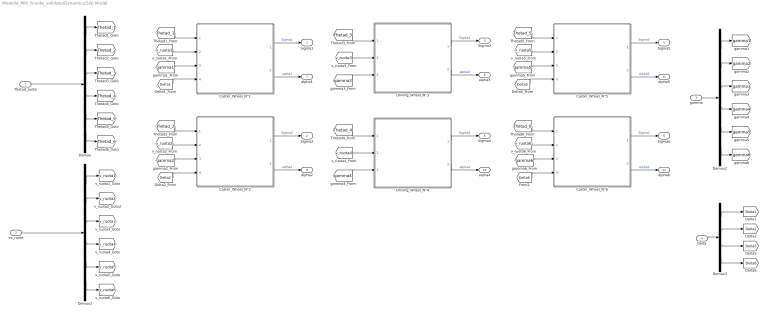
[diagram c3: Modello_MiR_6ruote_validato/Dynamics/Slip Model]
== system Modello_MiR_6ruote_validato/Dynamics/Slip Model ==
  Thetad_ruote : Inport
  vx_ruote : Inport  Port=2
  gamma : Inport  Port=3
  Delta : Inport  Port=4
  Caster_Wheel_N°1 : Subsystem
  Caster_Wheel_N°2 : Subsystem
  Caster_Wheel_N°5 : Subsystem
  Caster_Wheel_N°6 : Subsystem
  Demux : Demux  Outputs=6
  Demux1 : Demux  Outputs=6
  Demux2 : Demux  Outputs=6
  Demux3 : Demux
  Driving_Wheel_N°3 : Subsystem
  Driving_Wheel_N°4 : Subsystem
  Sigma1 : Outport  PortDimensions=1
  Sigma2 : Outport  Port=2  PortDimensions=1
  Sigma3 : Outport  Port=3  PortDimensions=1
  Sigma4 : Outport  Port=4  PortDimensions=1
  Sigma5 : Outport  Port=5  PortDimensions=1
  Sigma6 : Outport  Port=6  PortDimensions=1
  alpha1 : Outport  Port=7  PortDimensions=1
  alpha2 : Outport  Port=8  PortDimensions=1
  alpha3 : Outport  Port=9  PortDimensions=1
  alpha4 : Outport  Port=10  PortDimensions=1
  alpha5 : Outport  Port=11  PortDimensions=1
  alpha6 : Outport  Port=12  PortDimensions=1
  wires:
  Caster_Wheel_N°1/2(alpha1) -> alpha1/1  "alpha1"
  Demux/3 -> [Thetad_3]
  [Delta5] -> Caster_Wheel_N°5/4(Delta5)
  Demux1/1 -> [v_ruota1]
  Driving_Wheel_N°3/2(alpha3) -> alpha3/1  "alpha3"
  Demux1/6 -> [v_ruota6]
  Caster_Wheel_N°5/2(alpha5) -> alpha5/1  "alpha5"
  Demux1/2 -> [v_ruota2]
  Demux/1 -> [Thetad_1]
  Demux3/2 -> [Delta2]
  [v_ruota6] -> Caster_Wheel_N°6/2(vx_ruota6)
  Driving_Wheel_N°4/1(Sigma4) -> Sigma4/1  "Sigma4"
  Demux2/5 -> [gamma5]
  Caster_Wheel_N°6/2(alpha6) -> alpha6/1  "alpha2"
  Driving_Wheel_N°3/1(Sigma3) -> Sigma3/1  "Sigma3"
  [Thetad_1] -> Caster_Wheel_N°1/1(Thetad_1)
  Demux/2 -> [Thetad_2]
  Driving_Wheel_N°4/2(alpha4) -> alpha4/1  "alpha4"
  Demux1/4 -> [v_ruota4]
  Thetad_ruote/1 -> Demux/1
  [gamma6] -> Caster_Wheel_N°6/3(gamma6)
  Caster_Wheel_N°2/2(alpha2) -> alpha2/1  "alpha2"
  Caster_Wheel_N°5/1(Sigma5) -> Sigma5/1  "Sigma5"
  [v_ruota3] -> Driving_Wheel_N°3/2(vx_ruota3)
  Caster_Wheel_N°1/1(Sigma1) -> Sigma1/1  "Sigma1"
  [Thetad_4] -> Driving_Wheel_N°4/1(Thetad_4)
  Demux/5 -> [Thetad_5]
  Caster_Wheel_N°2/1(Sigma2) -> Sigma2/1  "Sigma2"
  [gamma1] -> Caster_Wheel_N°1/3(gamma1)
  Demux/4 -> [Thetad_4]
  [v_ruota4] -> Driving_Wheel_N°4/2(vx_ruota4)
  Demux3/1 -> [Delta1]
  Caster_Wheel_N°6/1(Sigma6) -> Sigma6/1  "Sigma2"
  Demux3/3 -> [Delta5]
  Demux/6 -> [Thetad_6]
  Demux2/6 -> [gamma6]
  [Thetad_5] -> Caster_Wheel_N°5/1(Thetad_5)
  [Delta1] -> Caster_Wheel_N°1/4(Delta1)
  Demux1/5 -> [v_ruota5]
  Delta/1 -> Demux3/1
  gamma/1 -> Demux2/1
  [Thetad_3] -> Driving_Wheel_N°3/1(Thetad_3)
  vx_ruote/1 -> Demux1/1
  Demux2/4 -> [gamma4]
  Demux2/1 -> [gamma1]
  Demux2/2 -> [gamma2]
  [v_ruota2] -> Caster_Wheel_N°2/2(vx_ruota2)
  [gamma5] -> Caster_Wheel_N°5/3(gamma5)
  Demux2/3 -> [gamma3]
  [gamma4] -> Driving_Wheel_N°4/3(gamma4)
  [Thetad_2] -> Caster_Wheel_N°2/1(Thetad_2)
  [v_ruota1] -> Caster_Wheel_N°1/2(vx_ruota1)
  [gamma2] -> Caster_Wheel_N°2/3(gamma2)
  Demux1/3 -> [v_ruota3]
  [Delta6] -> Caster_Wheel_N°6/4(Delta6)
  [Thetad_6] -> Caster_Wheel_N°6/1(Thetad_6)
  Demux3/4 -> [Delta6]
  [Delta2] -> Caster_Wheel_N°2/4(Delta2)
  [gamma3] -> Driving_Wheel_N°3/3(gamma3)
  [v_ruota5] -> Caster_Wheel_N°5/2(vx_ruota5)

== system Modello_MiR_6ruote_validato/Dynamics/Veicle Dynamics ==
  FL : Inport
  FT : Inport  Port=2
  M : Inport  Port=3
  Delta : Inport  Port=4
  Demux : Demux
  Integrator : Integrator
  Integrator1 : Integrator
  Integrator6 : Integrator
  Mux14 : Mux  Inputs=6
  Normal Reaction : Subsystem
  Rotation Dynamics : Subsystem
  Rotational Matrix : MATLAB Function  TreatAsAtomicUnit=on
  Scope : Scope
  Translation Dynamics : Subsystem
  Normal_react : Outport
  xd : Outport  Port=2  PortDimensions=1
  yd : Outport  Port=3  PortDimensions=1
  Psid : Outport  Port=4  PortDimensions=1
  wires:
  Normal Reaction/4(F43) -> Mux14/4  "F43"
  Demux/1 -> Normal Reaction/1(Delta1)
  Demux/2 -> Normal Reaction/2(Delta2)
  Normal Reaction/5(F53) -> Mux14/5  "F53"
  Demux/4 -> Normal Reaction/4(Delta6)
  Normal Reaction/1(F13) -> Mux14/1  "F13"
  Rotation Dynamics/1(Psidd) -> Integrator6/1
  Normal Reaction/2(F23) -> Mux14/2  "F23"
  Normal Reaction/6(F63) -> Mux14/6  "F63"
  Demux/3 -> Normal Reaction/3(Delta5)
  Normal Reaction/3(F33) -> Mux14/3  "F33"
  Integrator6/1 -> Psid/1, Translation Dynamics/5(Psid)  "Psid"
  Mux14/1 -> Scope/1, Normal_react/1
  Delta/1 -> Rotation Dynamics/2("Delta "), Demux/1, Rotational Matrix/3(Delta)
  Rotational Matrix/2(Fy_generalized) -> Rotation Dynamics/3(Fy_generalized), Translation Dynamics/2(Fy_generalized)
  FL/1 -> Rotational Matrix/1(FL)
  FT/1 -> Rotational Matrix/2(FT)
  Rotational Matrix/1(Fx_generalized) -> Rotation Dynamics/1(Fx_generalized), Translation Dynamics/1(Fx_generalized)
  Translation Dynamics/1(xdd) -> Integrator/1
  Translation Dynamics/2(ydd) -> Integrator1/1
  Integrator/1 -> Translation Dynamics/3(xd), xd/1
  Integrator1/1 -> Translation Dynamics/4(yd), yd/1
  M/1 -> Rotation Dynamics/4(M)
  Translation Dynamics/3(a_tau) -> Normal Reaction/5(a_tau)
  Translation Dynamics/4(a_n) -> Normal Reaction/6(a_n)

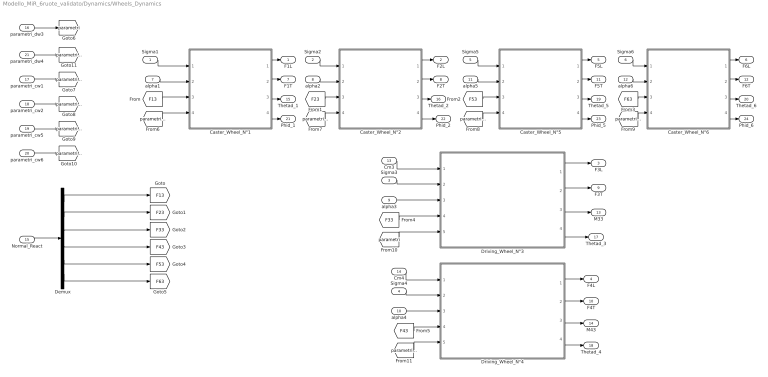
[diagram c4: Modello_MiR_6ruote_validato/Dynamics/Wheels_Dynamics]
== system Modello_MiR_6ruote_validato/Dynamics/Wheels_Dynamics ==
  Sigma1 : Inport
  Sigma2 : Inport  Port=2
  Sigma3 : Inport  Port=3
  Sigma4 : Inport  Port=4
  Sigma5 : Inport  Port=5
  Sigma6 : Inport  Port=6
  alpha1 : Inport  Port=7
  alpha2 : Inport  Port=8
  alpha3 : Inport  Port=9
  alpha4 : Inport  Port=10
  alpha5 : Inport  Port=11
  alpha6 : Inport  Port=12
  Cm3 : Inport  Port=13
  Cm4 : Inport  Port=14
  Normal_React : Inport  Port=15
  parametri_dw3 : Inport  Port=16
  parametri_cw1 : Inport  Port=17
  parametri_cw2 : Inport  Port=18
  parametri_cw5 : Inport  Port=19
  parametri_cw6 : Inport  Port=20
  parametri_dw4 : Inport  Port=21
  Caster_Wheel_N°1 : Subsystem
  Caster_Wheel_N°2 : Subsystem
  Caster_Wheel_N°5 : Subsystem
  Caster_Wheel_N°6 : Subsystem
  Demux : Demux  Outputs=6
  Driving_Wheel_N°3 : Subsystem
  Driving_Wheel_N°4 : Subsystem
  F1L : Outport  PortDimensions=1
  F2L : Outport  Port=2  PortDimensions=1
  F3L : Outport  Port=3  PortDimensions=1
  F4L : Outport  Port=4  PortDimensions=1
  F5L : Outport  Port=5  PortDimensions=1
  F6L : Outport  Port=6  PortDimensions=1
  F1T : Outport  Port=7  PortDimensions=1
  F2T : Outport  Port=8  PortDimensions=1
  F3T : Outport  Port=9  PortDimensions=1
  F4T : Outport  Port=10  PortDimensions=1
  F5T : Outport  Port=11  PortDimensions=1
  F6T : Outport  Port=12  PortDimensions=1
  M33 : Outport  Port=13  PortDimensions=1
  M43 : Outport  Port=14  PortDimensions=1
  Thetad_1 : Outport  Port=15  PortDimensions=1
  Thetad_2 : Outport  Port=16  PortDimensions=1
  Thetad_3 : Outport  Port=17  PortDimensions=1
  Thetad_4 : Outport  Port=18  PortDimensions=1
  Thetad_5 : Outport  Port=19  PortDimensions=1
  Thetad_6 : Outport  Port=20  PortDimensions=1
  Phid_1 : Outport  Port=21  PortDimensions=1
  Phid_2 : Outport  Port=22  PortDimensions=1
  Phid_5 : Outport  Port=23  PortDimensions=1
  Phid_6 : Outport  Port=24  PortDimensions=1
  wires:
  Sigma5/1 -> Caster_Wheel_N°5/1(Sigma5)
  Caster_Wheel_N°6/1(F6L) -> F6L/1
  Sigma2/1 -> Caster_Wheel_N°2/1(Sigma2)
  Caster_Wheel_N°6/3(Thetad_6) -> Thetad_6/1
  Caster_Wheel_N°2/1(F2L) -> F2L/1
  Caster_Wheel_N°6/4(Phid_6) -> Phid_6/1
  Caster_Wheel_N°5/3(Thetad_5) -> Thetad_5/1
  alpha1/1 -> Caster_Wheel_N°1/2(alpha1)
  Sigma1/1 -> Caster_Wheel_N°1/1(Sigma1)
  Caster_Wheel_N°1/2(F1T) -> F1T/1
  Caster_Wheel_N°1/4(Phid_1) -> Phid_1/1
  Caster_Wheel_N°5/2(F5T) -> F5T/1
  Caster_Wheel_N°5/4(Phid_5) -> Phid_5/1
  Caster_Wheel_N°5/1(F5L) -> F5L/1
  Caster_Wheel_N°6/2(F6T) -> F6T/1
  Sigma6/1 -> Caster_Wheel_N°6/1(Sigma6)
  alpha6/1 -> Caster_Wheel_N°6/2(alpha6)
  Caster_Wheel_N°2/4(Phid_2) -> Phid_2/1
  alpha5/1 -> Caster_Wheel_N°5/2(alpha5)
  Caster_Wheel_N°2/2(F2T) -> F2T/1
  Caster_Wheel_N°1/1(F1L) -> F1L/1
  alpha2/1 -> Caster_Wheel_N°2/2(alpha2)
  Caster_Wheel_N°2/3(Thetad_2) -> Thetad_2/1
  Caster_Wheel_N°1/3(Thetad_1) -> Thetad_1/1
  alpha4/1 -> Driving_Wheel_N°4/3(alpha4)
  alpha3/1 -> Driving_Wheel_N°3/3(alpha3)
  Driving_Wheel_N°4/2(F4T) -> F4T/1
  Driving_Wheel_N°3/3(M33) -> M33/1
  Driving_Wheel_N°4/4(Thetad_4) -> Thetad_4/1
  Sigma4/1 -> Driving_Wheel_N°4/2(Sigma4)
  Driving_Wheel_N°4/3(M43) -> M43/1
  Sigma3/1 -> Driving_Wheel_N°3/2(Sigma3)
  Driving_Wheel_N°3/1(F3L) -> F3L/1
  Cm3/1 -> Driving_Wheel_N°3/1(Cm3)
  Driving_Wheel_N°3/4(Thetad_3) -> Thetad_3/1
  Driving_Wheel_N°3/2(F3T) -> F3T/1
  Driving_Wheel_N°4/1(F4L) -> F4L/1
  Cm4/1 -> Driving_Wheel_N°4/1(Cm4)
  Normal_React/1 -> Demux/1
  [F13] -> Caster_Wheel_N°1/3(F13)
  [F23] -> Caster_Wheel_N°2/3(F23)
  [F53] -> Caster_Wheel_N°5/3(F53)
  [F63] -> Caster_Wheel_N°6/3(F63)
  [F33] -> Driving_Wheel_N°3/4(F33)
  [F43] -> Driving_Wheel_N°4/4(F43)
  Demux/1 -> [F13]
  Demux/2 -> [F23]
  Demux/3 -> [F33]
  Demux/4 -> [F43]
  Demux/5 -> [F53]
  Demux/6 -> [F63]
  parametri_dw3/1 -> [parametri]
  [parametri_cw1] -> Caster_Wheel_N°1/4(parametri_cw1)
  [parametri_cw2] -> Caster_Wheel_N°2/4(parametri)
  [parametri_cw5] -> Caster_Wheel_N°5/4(parametri)
  [parametri_cw6] -> Caster_Wheel_N°6/4(parametri)
  [parametri] -> Driving_Wheel_N°3/5(parametri_dw3)
  [parametri_dw4] -> Driving_Wheel_N°4/5(parametri_dw4)
  parametri_cw1/1 -> [parametri_cw1]
  parametri_cw2/1 -> [parametri_cw2]
  parametri_cw5/1 -> [parametri_cw5]
  parametri_cw6/1 -> [parametri_cw6]
  parametri_dw4/1 -> [parametri_dw4]

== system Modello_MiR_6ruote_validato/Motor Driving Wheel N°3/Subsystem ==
  Thetad_SET : Inport
  Thetad_FB : Inport  Port=2
  iFB : Inport  Port=3
  " 1" : slpidlib/PID Controller  Controller=PID  Form=Parallel  TimeDomain=Continuous-time  UseExternalTs=off  SampleTime=-1  IntegratorMethod=Forward Euler  FilterMethod=Forward Euler  ControllerParametersSource=internal  P=Kp_v  I=Ki_v  UseKiTs=off  D=0  N=1  UseFilter=on  TunerSelectOption=Transfer Function Based (PID Tuner App)  InitialConditionSource=internal  InitialConditionForIntegrator=0  InitialConditionForFilter=0  DifferentiatorICPrevScaledInput=0  ExternalReset=none  TrackingMode=off  Kt=1  LimitOutput=on  SatLimitsSource=internal  UpperSaturationLimit=iMax  LowerSaturationLimit=-iMax  LinearizeAsGain=on  AntiWindupMode=back-calculation  Kb=1  POutMin=[]  POutMax=[]  IOutMin=[]  IOutMax=[]  DOutMin=[]  DOutMax=[]  NOutMin=[]  NOutMax=[]  SumOutMin=[]  SumOutMax=[]  SaturationOutMin=[]  SaturationOutMax=[]  PParamMin=0  PParamMax=[]  IParamMin=0  IParamMax=[]  DParamMin=0  DParamMax=[]  NParamMin=[]  NParamMax=[]  KbParamMin=[]  KbParamMax=[]  KtParamMin=[]  KtParamMax=[]  KbOutMin=[]  KbOutMax=[]  KtOutMin=[]  KtOutMax=[]  IntegratorOutMin=[]  IntegratorOutMax=[]  FilterOutMin=[]  FilterOutMax=[]  SumI1OutMin=[]  SumI1OutMax=[]  SumI2OutMin=[]  SumI2OutMax=[]  SumI3OutMin=[]  SumI3OutMax=[]  SumI4OutMin=[]  SumI4OutMax=[]  SumDOutMin=[]  SumDOutMax=[]  DifferentiatorOutMin=[]  DifferentiatorOutMax=[]  FilterDiffOutCoefMin=[]  FilterDiffOutCoefMax=[]  ReciprocalOutMin=[]  ReciprocalOutMax=[]  SumDenOutMin=[]  SumDenOutMax=[]  SumNumOutMin=[]  SumNumOutMax=[]  DivideOutMin=[]  DivideOutMax=[]  UdiffTsProdOutMin=[]  UdiffTsProdOutMax=[]  NTsProdOutMin=[]  NTsProdOutMax=[]  UintegralTsProdOutMin=[]  UintegralTsProdOutMax=[]  UngainTsProdOutMin=[]  UngainTsProdOutMax=[]  IntegratorContinuousStateAttributes=''  IntegratorStateMustResolveToSignalObject=off  IntegratorRTWStateStorageClass=Auto  FilterContinuousStateAttributes=''  FilterStateMustResolveToSignalObject=off  FilterRTWStateStorageClass=Auto  ParallelPVariant=InternalParameters  IdealPVariant=Disabled  IVariant=InternalParameters  DVariant=InternalParameters  IntegratorVariant=Continuous  SatVariant=Enabled  AWVariant=BackCalculation  PCopyVariant=Disabled  TRVariant=Disabled  FdbkBlocksVariant=Forward  IdealPFdbkVariant=Disabled  SatFdbkVariant=Disabled  DerivativeFilterVariant=ContFilter  NVariant=InternalParameters  NCopyVariant=Disabled  FilterICVariant=InternalICsFilter  IntegratorICVariant=InternalICs  ExternalResetVariant=Disabled  TRSumVariant=Passthrough  SumFdbkVariant=Disabled  SumVariant=Sum_PID  TsampFilterVariant=InternalTs  TsampNgainVariant=Passthrough  TsampIntegralVariant=Passthrough  ExternalSaturationOutDataTypeStr=Inherit: Same as second input  aMode=0
  PID Controller2 : slpidlib/PID Controller  Controller=PID  Form=Parallel  TimeDomain=Continuous-time  UseExternalTs=off  SampleTime=-1  IntegratorMethod=Forward Euler  FilterMethod=Forward Euler  ControllerParametersSource=internal  P=Kp_i  I=Ki_i  UseKiTs=off  D=0  N=100  UseFilter=on  TunerSelectOption=Transfer Function Based (PID Tuner App)  InitialConditionSource=internal  InitialConditionForIntegrator=0  InitialConditionForFilter=0  DifferentiatorICPrevScaledInput=0  ExternalReset=none  TrackingMode=off  Kt=1  LimitOutput=on  SatLimitsSource=internal  UpperSaturationLimit=VaMax  LowerSaturationLimit=-VaMax  LinearizeAsGain=on  AntiWindupMode=back-calculation  Kb=1  POutMin=[]  POutMax=[]  IOutMin=[]  IOutMax=[]  DOutMin=[]  DOutMax=[]  NOutMin=[]  NOutMax=[]  SumOutMin=[]  SumOutMax=[]  SaturationOutMin=[]  SaturationOutMax=[]  PParamMin=[]  PParamMax=[]  IParamMin=[]  IParamMax=[]  DParamMin=[]  DParamMax=[]  NParamMin=[]  NParamMax=[]  KbParamMin=[]  KbParamMax=[]  KtParamMin=[]  KtParamMax=[]  KbOutMin=[]  KbOutMax=[]  KtOutMin=[]  KtOutMax=[]  IntegratorOutMin=[]  IntegratorOutMax=[]  FilterOutMin=[]  FilterOutMax=[]  SumI1OutMin=[]  SumI1OutMax=[]  SumI2OutMin=[]  SumI2OutMax=[]  SumI3OutMin=[]  SumI3OutMax=[]  SumI4OutMin=[]  SumI4OutMax=[]  SumDOutMin=[]  SumDOutMax=[]  DifferentiatorOutMin=[]  DifferentiatorOutMax=[]  FilterDiffOutCoefMin=[]  FilterDiffOutCoefMax=[]  ReciprocalOutMin=[]  ReciprocalOutMax=[]  SumDenOutMin=[]  SumDenOutMax=[]  SumNumOutMin=[]  SumNumOutMax=[]  DivideOutMin=[]  DivideOutMax=[]  UdiffTsProdOutMin=[]  UdiffTsProdOutMax=[]  NTsProdOutMin=[]  NTsProdOutMax=[]  UintegralTsProdOutMin=[]  UintegralTsProdOutMax=[]  UngainTsProdOutMin=[]  UngainTsProdOutMax=[]  IntegratorContinuousStateAttributes=''  IntegratorStateMustResolveToSignalObject=off  IntegratorRTWStateStorageClass=Auto  FilterContinuousStateAttributes=''  FilterStateMustResolveToSignalObject=off  FilterRTWStateStorageClass=Auto  ParallelPVariant=InternalParameters  IdealPVariant=Disabled  IVariant=InternalParameters  DVariant=InternalParameters  IntegratorVariant=Continuous  SatVariant=Enabled  AWVariant=BackCalculation  PCopyVariant=Disabled  TRVariant=Disabled  FdbkBlocksVariant=Forward  IdealPFdbkVariant=Disabled  SatFdbkVariant=Disabled  DerivativeFilterVariant=ContFilter  NVariant=InternalParameters  NCopyVariant=Disabled  FilterICVariant=InternalICsFilter  IntegratorICVariant=InternalICs  ExternalResetVariant=Disabled  TRSumVariant=Passthrough  SumFdbkVariant=Disabled  SumVariant=Sum_PID  TsampFilterVariant=InternalTs  TsampNgainVariant=Passthrough  TsampIntegralVariant=Passthrough  ExternalSaturationOutDataTypeStr=Inherit: Same as second input  aMode=0
  Scope : Scope
  Scope1 : Scope
  Scope2 : Scope
  Scope3 : Scope  NumInputPorts=2
  Sum1 : Sum  Inputs=|+-
  Sum2 : Sum  Inputs=|+-
  VaRif : Outport  VectorParamsAs1DForOutWhenUnconnected=off
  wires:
  Thetad_FB/1 -> Scope3/2, Sum1/2
  " 1"/1 -> Scope2/1, Sum2/1
  PID Controller2/1 -> Scope1/1, VaRif/1
  iFB/1 -> Sum2/2
  Thetad_SET/1 -> Scope3/1, Sum1/1
  Sum1/1 -> " 1"/1, Scope/1
  Sum2/1 -> PID Controller2/1

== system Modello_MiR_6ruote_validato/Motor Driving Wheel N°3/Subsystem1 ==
  VaRif : Inport
  Thetad_FB : Inport  Port=2
  Add : Sum  Inputs=+--
  Gain : Gain  Gain=rap_rid
  Gain1 : Gain  Gain=1/L
  Gain2 : Gain  Gain=Kc
  Gain3 : Gain  Gain=R
  Gain4 : Gain  Gain=Kc
  Integrator : Integrator
  Scope : Scope
  Scope1 : Scope
  Torque Cm : Outport  VectorParamsAs1DForOutWhenUnconnected=off
  iFB : Outport  Port=2  VectorParamsAs1DForOutWhenUnconnected=off
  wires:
  VaRif/1 -> Add/1
  Add/1 -> Gain1/1
  Gain1/1 -> Integrator/1
  Integrator/1 -> Gain4/1, iFB/1, Gain3/1
  Gain3/1 -> Add/3
  Gain4/1 -> Scope1/1, Gain/1
  Thetad_FB/1 -> Gain2/1, Scope/1
  Gain2/1 -> Add/2
  Gain/1 -> Torque Cm/1
